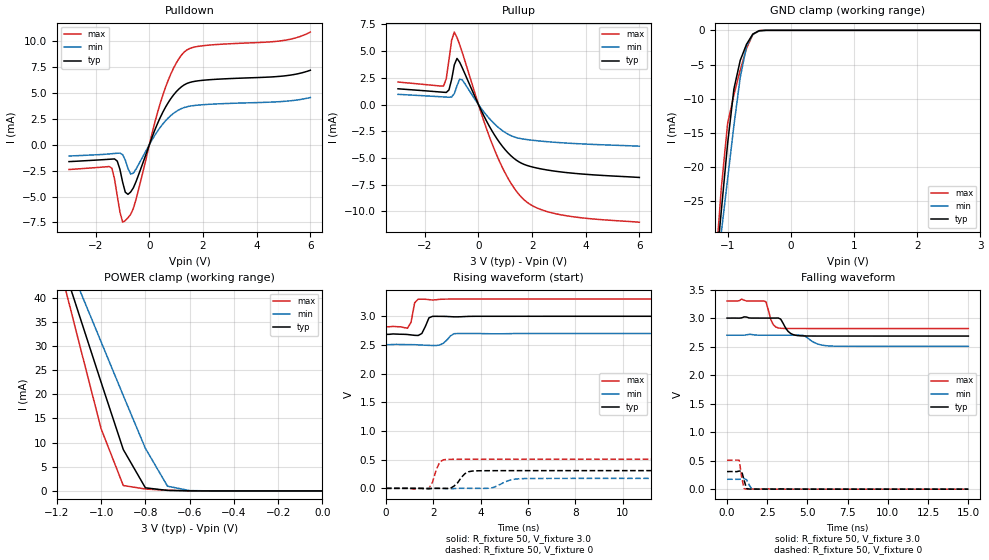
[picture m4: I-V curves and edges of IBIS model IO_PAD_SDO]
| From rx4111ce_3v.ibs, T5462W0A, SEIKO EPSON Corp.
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[Model]   IO_PAD_SDO
Model_type 3-state
Enable Active-High
Polarity Non-Inverting
Vmeas=1.50
C_comp   2.5p   2.0p   3.0p
[Temperature Range] 25   105   -40
[Voltage Range]   3.0   2.7   3.3
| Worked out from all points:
|   slope of the pulldown table from 0 to 0.45 V, typ, clamps not added: 158 ohm
|   slope of the pullup table from 0 to 0.45 V, typ, clamps not added: 202 ohm
|   GND clamp passes 1 mA (typ) near -0.63 V on its own axis
|   POWER clamp passes 1 mA (typ) near -0.80 V on its own axis
|   falling waveform, R_fixture 50, V_fixture 3.0: 20-80 % time 451ps typ, 699ps min, 320ps max; typ from 3 V to 2.69 V
|   falling waveform, R_fixture 50, V_fixture 0: 20-80 % time 184ps typ, 207ps min, 183ps max; typ from 0.309 V to 0 V
|   rising waveform, R_fixture 50, V_fixture 3.0: 20-80 % time 208ps typ, 275ps min, 129ps max; typ from 2.69 V to 3 V
|   rising waveform, R_fixture 50, V_fixture 0: 20-80 % time 380ps typ, 554ps min, 259ps max; typ from 0 V to 0.309 V
[Pullup]
-3V       1.471mA    952.3uA    2.104mA
-1.3V     1.147mA    709.6uA    1.738mA
-1.2V     1.13mA     694.3uA    2.414mA
-1.1V     1.366mA    678.8uA    4.16mA
-1V       2.339mA    705.3uA    6.008mA
-900mV    3.706mA    1.017mA    6.776mA
-800mV    4.313mA    1.748mA    6.271mA
-600mV    3.419mA    2.299mA    4.848mA
600mV     -2.854mA   -1.818mA   -4.245mA
1.6V      -5.487mA   -3.2mA     -8.66mA
2.9V      -6.251mA   -3.543mA   -10.23mA
6V        -6.822mA   -3.898mA   -11.01mA
[Pulldown]
-3V       -1.645mA   -1.105mA   -2.403mA
-1.4V     -1.401mA   -881.9uA   -2.281mA
-1.2V     -1.594mA   -838.1uA   -4.933mA
-1V       -3.61mA    -971.9uA   -7.471mA
-800mV    -4.792mA   -2.307mA   -7.046mA
-600mV    -4.172mA   -2.75mA    -6.157mA
500mV     3.111mA    1.977mA    4.757mA
900mV     4.773mA    3.002mA    7.349mA
1.3V      5.744mA    3.563mA    8.902mA
2V        6.182mA    3.832mA    9.508mA
5V        6.594mA    4.15mA     10.01mA
6V        7.147mA    4.525mA    10.82mA
[GND Clamp]
-3V       -218.9mA   -181.8mA   -264.5mA
-1.2V     -36.43mA   -37.5mA    -35.6mA
-1.1V     -26.48mA   -29.64mA   -23.15mA
-1V       -16.59mA   -21.78mA   -13.65mA
-900mV    -8.58mA    -13.93mA   -9.45mA
-800mV    -4.393mA   -6.884mA   -5.813mA
-700mV    -2.03mA    -2.311mA   -2.637mA
-600mV    -545.2uA   -558.8uA   -605.7uA
-500mV    -56.87uA   -90.58uA   -35.51uA
3V        59.8pA     61.22nA    50.02pA
[POWER Clamp]
-3V       306.9mA    255.3mA    375.5mA
-1.2V     50.66mA    53.08mA    48.75mA
-1.1V     36.55mA    41.95mA    30.73mA
-1V       22.47mA    30.83mA    12.85mA
-900mV    8.574mA    19.75mA    1.117mA
-800mV    640.7uA    8.813mA    397uA
-700mV    110.3uA    975.9uA    130.4uA
-600mV    21.48uA    71.72uA    21uA
0V        59.8pA     538.2pA    58.66pA
[Falling Waveform]
R_fixture=50
V_fixture=3.0
V_fixture_min=2.7
V_fixture_max=3.3
0s        3V         2.7V       3.3V
909.1ps   3.004V     2.699V     3.333V
2.424ns   3V         2.7V       3.285V
2.727ns   3V         2.7V       2.969V
2.879ns   3V         2.7V       2.883V
3.333ns   2.983V     2.7V       2.821V
3.788ns   2.769V     2.7V       2.818V
4.394ns   2.693V     2.7V       2.817V
6.364ns   2.685V     2.511V     2.817V
15ns      2.685V     2.505V     2.817V
[Falling Waveform]
R_fixture=50
V_fixture=0
V_fixture_min=0
V_fixture_max=0
0s        308.8mV    173.5mV    508.3mV
606.1ps   306.9mV    172.1mV    509.7mV
757.6ps   318mV      172.6mV    508.3mV
909.1ps   317mV      178mV      216.5mV
1.061ns   157.9mV    186.3mV    9.726mV
1.212ns   11.24mV    166.1mV    1.678mV
1.364ns   2.61mV     80.05mV    1.351mV
1.515ns   995.9uV    13.81mV    1.269mV
1.818ns   738uV      1.359mV    1.133mV
15ns      8.88uV     8.785uV    8.947uV
[Rising Waveform]
R_fixture=50
V_fixture=3.0
V_fixture_min=2.7
V_fixture_max=3.3
0s        2.685V     2.505V     2.816V
909.1ps   2.683V     2.506V     2.791V
1.061ns   2.675V     2.505V     2.894V
1.212ns   2.667V     2.504V     3.233V
1.364ns   2.665V     2.502V     3.298V
1.515ns   2.699V     2.498V     3.298V
1.818ns   2.973V     2.493V     3.29V
1.97ns    2.999V     2.491V     3.284V
3.03ns    2.99V      2.699V     3.3V
15ns      3V         2.7V       3.3V
[Rising Waveform]
R_fixture=50
V_fixture=0
V_fixture_min=0
V_fixture_max=0
0s        0V         0V         0V
1.818ns   -8.941mV   101.6uV    1.029mV
2.273ns   -401.8uV   -719.8uV   458.1mV
2.576ns   -2.343mV   -3.614mV   504.1mV
2.879ns   40.19mV    -4.396mV   506.2mV
3.333ns   254.5mV    2.07uV     507.1mV
3.788ns   304.8mV    -561.4uV   507.4mV
4.545ns   307.8mV    15.86mV    507.6mV
5.758ns   308.4mV    169.1mV    507.9mV
15ns      308.8mV    173.4mV    508.3mV
[Ramp]
R_load=50
dV/dt_r   1.853E-1/3.602E-10   1.041E-1/5.454E-10   3.050E-1/2.297E-10
dV/dt_f   1.891E-1/4.324E-10   1.172E-1/6.934E-10   2.901E-1/2.863E-10
|[End   IO_PAD_SDO
